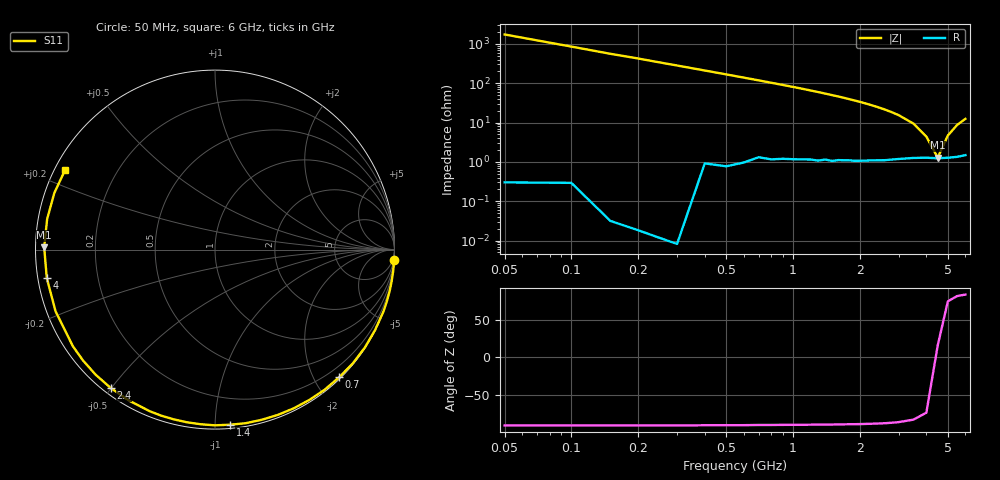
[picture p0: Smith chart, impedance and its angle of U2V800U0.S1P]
! SIEMENS Discrete & RF Semiconductors
! BBY52-02W
! Si Tuning Diode in SCD-80
! VR = 0.8 V
! S-Parameters:  September  1997
# GHz  S  MA  R  50
!  f  S11
! GHz  MAG  ANG
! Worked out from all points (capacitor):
!   34 points, 50 MHz to 6 GHz, reference 50 ohm
!   read as one part to ground: C = 1.86 pF near 50 MHz
!   lowest |Z| = 1.28 ohm at 4.5 GHz (marker M1)
!   series resonance near 4.462 GHz, so ESL is about 680 pH
!   S11 on the Smith chart (normalised r, x): 50 MHz: 0, -35; 700 MHz: 0.03, -2.37; 1.4 GHz: 0.02, -1.09; 2.4 GHz: 0.02, -0.50; 4 GHz: 0.03, -0.08; 6 GHz: 0.03, +0.25
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0.05  1 -3.3
0.2  1 -13.4
0.3  1 -20.1
0.4  0.998 -26.7
0.5  0.9975 -33.2
0.6  0.9956 -39.6
0.7  0.9921 -45.8
0.8  0.9911 -52.0
0.9  0.9888 -57.9
1  0.9871 -63.6
1.1  0.9852 -69.2
1.3  0.9823 -80.0
1.4  0.9793 -85.1
1.5  0.979 -90.1
1.6  0.9763 -94.7
1.8  0.9732 -103.7
2  0.9711 -112.0
2.2  0.968 -119.8
2.4  0.9654 -127.0
2.6  0.9633 -133.7
2.8  0.9603 -140.0
3  0.9576 -145.8
3.5  0.9524 -158.9
4  0.9506 -170.4
4.5  0.9518 179.2
5  0.9506 169.7
5.5  0.9492 160.6
6  0.9456 152.2
